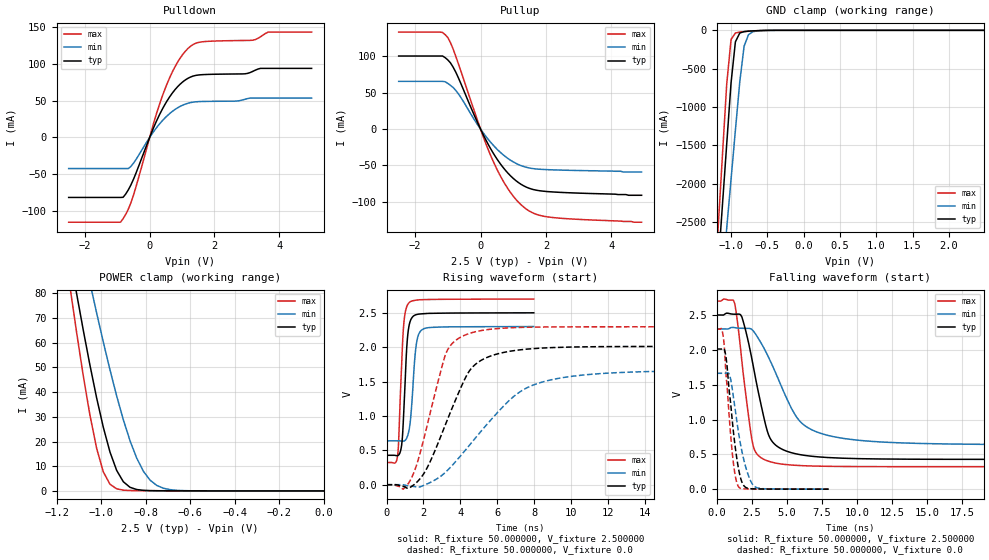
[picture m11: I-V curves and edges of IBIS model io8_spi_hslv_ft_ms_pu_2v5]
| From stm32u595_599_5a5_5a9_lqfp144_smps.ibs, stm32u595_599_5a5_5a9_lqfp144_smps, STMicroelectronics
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|   Model io8_spi_hslv_ft_ms_pu_2v5
[Model]  io8_spi_hslv_ft_ms_pu_2v5
Model_type I/O
Polarity   Non-Inverting
Enable   Active-Low
Vinl =   0.750000V
Vinh =   1.750000V
Vmeas =  1.250000V
Cref =   50.000000pF
Rref =   100.000000M
Vref =   0.0V
C_comp   3.438200pF   3.436700pF   3.473300pF
[Temperature Range]   25.000000   0.140000k   -40.000000
[Pullup Reference]   2.500000V   2.300000V   2.700000V
[Pulldown Reference]   0.0V   0.0V   0.0V
[POWER Clamp Reference]   2.500000V   2.300000V   2.700000V
[GND Clamp Reference]   0.0V   0.0V   0.0V
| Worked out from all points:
|   slope of the pulldown table from 0 to 0.375 V, typ, clamps not added: 10.1 ohm
|   slope of the pullup table from 0 to 0.375 V, typ, clamps not added: 11.7 ohm
|   GND clamp passes 1 mA (typ) near -0.50 V on its own axis
|   POWER clamp passes 1 mA (typ) near -0.85 V on its own axis
|   rising waveform, R_fixture 50.000000, V_fixture 2.500000: 20-80 % time 226ps typ, 272ps min, 222ps max; typ from 0.428 V to 2.5 V
|   rising waveform, R_fixture 50.000000, V_fixture 0.0: 20-80 % time 1.91ns typ, 3.39ns min, 1.31ns max; typ from 0 V to 2.01 V
|   falling waveform, R_fixture 50.000000, V_fixture 2.500000: 20-80 % time 1.3ns typ, 2.44ns min, 854ps max; typ from 2.5 V to 0.428 V
|   falling waveform, R_fixture 50.000000, V_fixture 0.0: 20-80 % time 657ps typ, 862ps min, 536ps max; typ from 2.01 V to 0 V
[Pulldown]
|Voltage   I(typ)   I(min)   I(max)
-2.5V     -81.61mA   -42.31mA   -115.3mA
-900mV    -81.61mA   -42.31mA   -115.3mA
-820mV    -81.42mA   -42.31mA   -110.6mA
-500mV    -56.95mA   -35.08mA   -78.57mA
140mV     15.18mA    9.02mA     22.02mA
460mV     44mA       25.98mA    64.37mA
860mV     68.91mA    40.27mA    102.2mA
1.26V     82.21mA    47.42mA    124mA
1.66V     85.53mA    48.99mA    130.3mA
3.18V     89.84mA    53.63mA    132.3mA
3.66V     94mA       53.63mA    143.4mA
5V        94mA       53.63mA    143.4mA
[Pullup]
|Voltage   I(typ)   I(min)   I(max)
-2.5V     100.4mA    65.58mA    133.3mA
-1.24V    100.4mA    65.58mA    133.3mA
-1V       95.05mA    62.84mA    125.9mA
-760mV    78.59mA    53.36mA    100.6mA
-40mV     3.893mA    2.628mA    5.181mA
360mV     -30.97mA   -20.78mA   -41.56mA
600mV     -47.45mA   -31.77mA   -63.92mA
840mV     -60.71mA   -40.52mA   -82.21mA
1.32V     -78.06mA   -51.54mA   -107.3mA
1.64V     -83.42mA   -54.54mA   -116.1mA
2.12V     -86.16mA   -55.91mA   -121.1mA
4.92V     -91mA      -59mA      -128mA
[GND_clamp]
|Voltage   I(typ)   I(min)   I(max)
-2.5V     -9.641A    -9.693A    -9.352A
-1.18V    -3.114A    -3.874A    -2.614A
-1.12V    -2.301A    -3.23A     -1.656A
-1.06V    -1.489A    -2.587A    -706.2mA
-1V       -685.8mA   -1.945A    -119.3mA
-940mV    -149.7mA   -1.304A    -34.73mA
-880mV    -35.54mA   -672.6mA   -23.06mA
-820mV    -16.19mA   -206.4mA   -17.27mA
-760mV    -10.58mA   -57.55mA   -12.41mA
-700mV    -7.152mA   -18.74mA   -8.24mA
-400mV    -103.3uA   -378.5uA   -41.74uA
2.48V     0A         13.22nA    0A
[POWER_clamp]
|Voltage   I(typ)   I(min)   I(max)
-2.49V    881.1mA    773.1mA    1.07A
-1.14V    95.32mA    122.8mA    82.93mA
-1.11V    79.97mA    109.7mA    64.26mA
-1.05V    50.95mA    84.3mA     30.69mA
-1.02V    37.7mA     72.08mA    17.29mA
-990mV    25.79mA    60.29mA    7.738mA
-930mV    8.312mA    38.47mA    853.1uA
-900mV    3.712mA    28.81mA    313.6uA
-840mV    566.2uA    13.29mA    123.7uA
-780mV    119.1uA    4.365mA    94.04uA
-660mV    38.99uA    251.5uA    57.77uA
0V        0A         18.93nA    0A
[Ramp]
| variable   typ   min   max
dV/dt_r  1.20644/1.90597n   0.99765/3.39056n   1.37763/1.30637n
dV/dt_f  1.24313/1.30328n   0.99709/2.43104n   1.42607/0.85081n
R_load = 50.000000
[Rising Waveform]
R_fixture= 50.000000
V_fixture= 2.500000
V_fixture_min= 2.300000
V_fixture_max= 2.700000
|time   V(typ)   V(min)   V(max)
0s        428.1mV    638.2mV    323.2mV
592.6ps   422.4mV    638.2mV    408.3mV
656.7ps   431.9mV    638.1mV    632mV
800.8ps   544.8mV    635.6mV    1.63V
961ps     1.219V     637mV      2.41V
1.089ns   1.966V     676mV      2.586V
1.201ns   2.284V     770.8mV    2.641V
1.586ns   2.471V     1.984V     2.683V
1.89ns    2.485V     2.247V     2.691V
7.976ns   2.5V       2.3V       2.7V
[Rising Waveform]
R_fixture= 50.000000
V_fixture= 0.0
V_fixture_min= 0.0
V_fixture_max= 0.0
|time   V(typ)   V(min)   V(max)
0s        470.3uV    553.8uV    445.9uV
1.001ns   -32.5mV    -6.418mV   -41.58mV
1.502ns   3.476mV    -26.26mV   189.9mV
1.902ns   116mV      -21.59mV   543.2mV
3.303ns   949.2mV    209.7mV    1.96V
4.404ns   1.619V     545.6mV    2.192V
5.205ns   1.821V     804.2mV    2.245V
7.608ns   1.972V     1.409V     2.29V
11.31ns   2.007V     1.611V     2.296V
49.85ns   2.011V     1.663V     2.296V
[Falling Waveform]
R_fixture= 50.000000
V_fixture= 2.500000
V_fixture_min= 2.300000
V_fixture_max= 2.700000
|time   V(typ)   V(min)   V(max)
0s        2.5V       2.3V       2.7V
1.201ns   2.512V     2.321V     2.711V
1.401ns   2.512V     2.315V     2.534V
1.802ns   2.473V     2.309V     1.841V
2.603ns   1.778V     2.275V     626mV
3.504ns   915.5mV    1.974V     416.2mV
4.004ns   673.8mV    1.762V     384.2mV
6.106ns   490.6mV    941.1mV    337.7mV
9.51ns    441.8mV    715.8mV    325.4mV
49.85ns   428.1mV    638.2mV    323.2mV
[Falling Waveform]
R_fixture= 50.000000
V_fixture= 0.0
V_fixture_min= 0.0
V_fixture_max= 0.0
|time   V(typ)   V(min)   V(max)
0s        2.011V     1.663V     2.296V
400.4ps   2.013V     1.663V     2.275V
528.5ps   2.016V     1.663V     2.1V
640.6ps   1.935V     1.663V     1.759V
912.9ps   1.392V     1.647V     1.014V
1.169ns   887.5mV    1.369V     429.8mV
1.57ns    289.7mV    808mV      34.82mV
2.178ns   16.07mV    250.4mV    3.523mV
2.771ns   4.061mV    30.46mV    2.165mV
7.976ns   470.3uV    553.8uV    445.9uV
